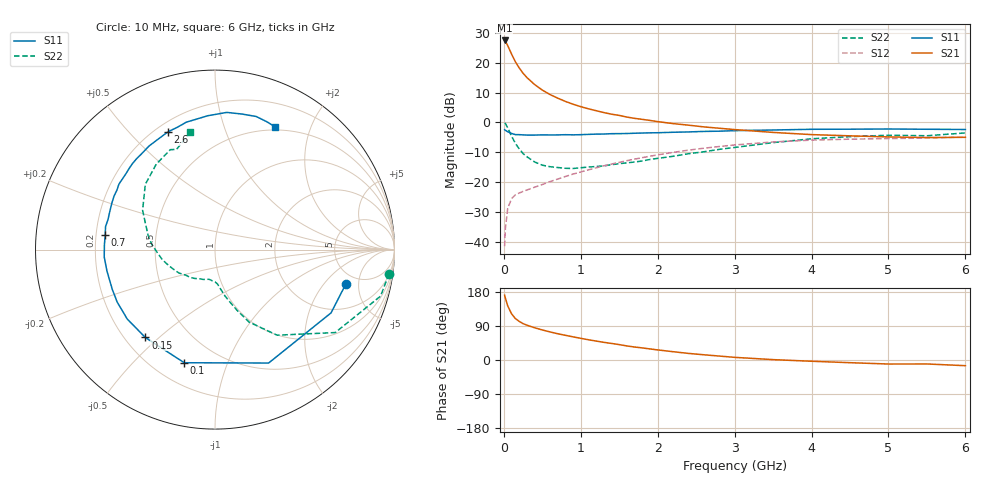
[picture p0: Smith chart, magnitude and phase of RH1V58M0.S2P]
! SIEMENS Small Signal Semiconductors
! BFR106
! Si NPN RF Bipolar Junction Transistor in SOT23
! VCE = 1.5 V  IC = 8 mA
! Common Emitter S-Parameters:  August  1996
# GHz  S  MA  R  50
!  f  S11  S21  S12  S22
! GHz  MAG  ANG  MAG  ANG  MAG  ANG  MAG  ANG
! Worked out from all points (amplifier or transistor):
!   36 points, 10 MHz to 6 GHz, reference 50 ohm
!   highest |S21| = 27.5 dB at 10 MHz (marker M1)
!   |S21| within 3 dB of that: start of sweep to 72.92 MHz
!   unconditionally stable (mu >= 1): 511.6 MHz to 2.486 GHz; 4.29 GHz to end of sweep
!   at 250 MHz: K = 0.65, MSG = 19.8 dB, |S12| = -23.1 dB
!   at 1.4 GHz: K = 1.12, MAG = 6.2 dB, |S12| = -14.0 dB
!   at 6 GHz: K = 1.03, MAG = -1.1 dB, |S12| = -4.9 dB
!   S11 on the Smith chart (normalised r, x): 10 MHz: 3.98, -3.49; 100 MHz: 0.32, -0.71; 150 MHz: 0.28, -0.45; 700 MHz: 0.24, +0.06; 2.6 GHz: 0.25, +0.65; 6 GHz: 0.46, +1.51
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0.01  0.7544 -14.5  23.73 171.0  0.0084 83.3  0.9792 -7.9
0.02  0.7365 -28.6  23.18 163.5  0.0166 76.2  0.9581 -15.7
0.05  0.6991 -64.7  19.54 142.9  0.0359 60.0  0.814 -34.6
0.1  0.6532 -105.2  14.05 122.1  0.0527 47.2  0.5894 -54.0
0.15  0.6248 -128.4  10.41 109.4  0.0609 40.8  0.4465 -64.8
0.2  0.6235 -141.7  8.215 101.9  0.0654 40.0  0.3605 -70.0
0.25  0.6183 -151.9  6.69 96.0  0.0698 40.0  0.3003 -74.4
0.3  0.6137 -158.9  5.66 91.9  0.0736 41.4  0.2656 -77.7
0.4  0.6137 -168.9  4.327 85.1  0.0819 44.5  0.2174 -82.5
0.5  0.6185 -176.2  3.489 79.3  0.0909 47.1  0.1918 -85.9
0.6  0.6167 177.6  2.94 74.1  0.1018 49.7  0.1809 -89.6
0.7  0.6173 172.2  2.555 69.3  0.1121 51.9  0.1753 -94.4
0.9  0.6191 164.3  2.02 61.1  0.136 54.4  0.1689 -102.3
1.1  0.6304 155.7  1.693 53.4  0.1603 55.4  0.1785 -111.3
1.3  0.6388 148.9  1.464 46.6  0.187 55.4  0.1869 -120.2
1.6  0.6522 139.4  1.229 37.1  0.2286 54.1  0.21 -134.0
2.2  0.6843 122.4  0.956 21.9  0.3146 47.5  0.2704 -160.1
2.6  0.7067 111.7  0.842 13.8  0.3694 41.5  0.3218 -176.9
3.5  0.7468 93.1  0.68 1.0  0.4708 26.3  0.4586 151.6
4.5  0.7702 78.6  0.596 -7.1  0.524 10.0  0.5778 124.5
5.5  0.7683 67.7  0.558 -10.5  0.5472 0.2  0.598 111.0
6  0.7615 63.8  0.563 -15.0  0.5697 -6.9  0.6672 102.0
